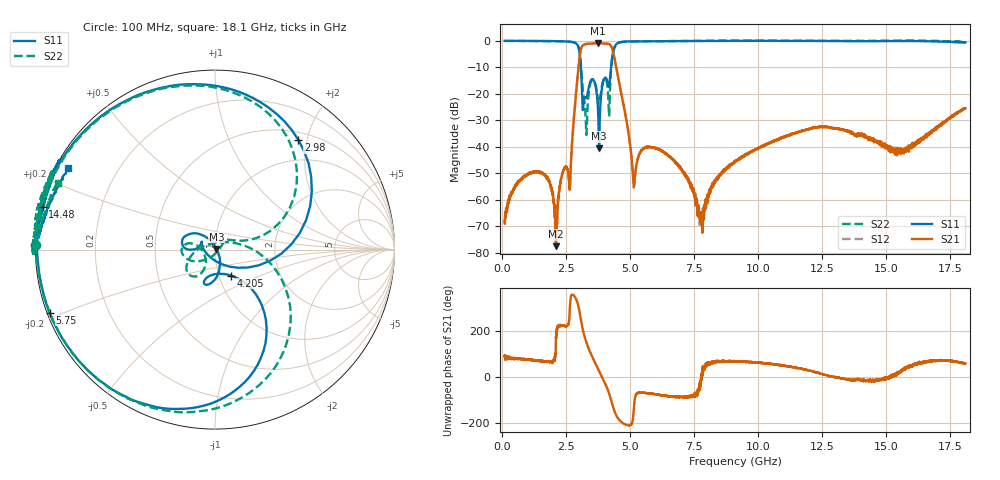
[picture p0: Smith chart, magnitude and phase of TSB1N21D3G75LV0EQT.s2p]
! TSB1N21D3G75LV0EQT  S-PARAMETER MODEL  ( General Type )
! Model Generated by TAIYO YUDEN Corporation (https://www.yuden.co.jp/en/)
! Version 1.0
! TAIYO YUDEN Control No. 20240527
! Copyright(c) 2024 TAIYO YUDEN CO.,LTD. All Rights Reserved.
! Products Name : Ceramic RF Devices
! Characteristics :
!  Passband freq : 3300-4200MHz ( At Passband , Insertion Loss : 2.0dB , VSWR 2.0 ),
!  Attenuation : 35 dB min at 600 to 2700MHz, 20 dB min at 4900 to 5900MHz, Impedance : 50 Ohm ,
!  Case Size : 2 x 1.25 / 0.079 x 0.049 [mm/inch] , Thickness : 0.65/ 0.026 [mm/inch]
!  (Conditions: Temperature = 25 degC , DC Bias Current/Voltage = 0A / 0V)
! External Node Assignments :
!  1  o---|-------|---o  2
!  |  BPF  |
! GND o---|-------|---o GND
! Frequency Range : 100MHz  -  18.1GHz  [ 3601 STEP ]
# MHZ S RI R 50
! Freq[MHz].  S11 Real  S11 Imag  S21 Real  S21 Imag  S12 Real  S12 Imag  S22 Real  S22 Imag
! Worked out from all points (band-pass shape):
!   3601 points, 100 MHz to 18.1 GHz, reference 50 ohm
!   highest |S21| = -0.80 dB at 3.755 GHz (marker M1); lowest = -77.6 dB at 2.105 GHz (marker M2)
!   |S21| within 3 dB of the highest: 3.069 GHz to 4.326 GHz (1.258 GHz wide, 34 % of centre)
!   lowest |S11| = -40.6 dB at 3.79 GHz (marker M3), VSWR 1.02, Z = 50.8 + j0.418 ohm
!   |S11| at or under -10 dB: 3.079 GHz to 4.255 GHz (1.176 GHz wide, 32.1 % of centre)
!   |S22| runs from -35.6 to 0.2 dB; largest |S21 - S12| = 0.0036
!   S11 on the Smith chart (normalised r, x): 100 MHz: -0.00, +0.01; 2.98 GHz: 0.62, +1.85; 4.205 GHz: 1.14, -0.34; 5.75 GHz: 0.01, -0.18; 14.48 GHz: 0.01, +0.12; 18.1 GHz: 0.04, +0.26
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100  -1.001 0.0239  -1.71e-06 0.000384  7.33e-05 0.000373  -0.9975 0.0244
1360  -0.9507 0.2975  0.00103 0.00315  0.00102 0.00318  -0.9471 0.2932
2105  -0.8359 0.5301  -0.000132 7.2e-06  -0.000195 7.2e-05  -0.8405 0.5139
2365  -0.7336 0.6551  -0.00225 -0.0023  -0.00224 -0.00226  -0.7472 0.6329
2650  -0.4868 0.8342  0.000983 -0.00133  0.000871 -0.00136  -0.526 0.8078
2980  0.4647 0.6114  0.1941 -0.2235  0.194 -0.2234  0.3388 0.7161
3100  0.1846 -0.0996  -0.3874 -0.628  -0.387 -0.6282  0.2688 0.0803
3260  -0.0725 0.0428  -0.8324 0.2452  -0.8326 0.2453  0.0353 0.0191
3435  -0.1618 0.00448  -0.306 0.8343  -0.3054 0.8343  -0.1345 -0.0622
3755  -0.0143 0.0391  0.7514 0.5172  0.7512 0.5167  -0.0739 -0.00109
3790  0.00833 0.00411  0.8158 0.4069  0.8159 0.4068  -0.0595 -0.0283
4205  0.089 -0.1446  0.1427 -0.847  0.1426 -0.8464  0.0688 0.0411
4520  -0.1974 -0.8875  -0.2228 -0.000711  -0.2227 -0.000543  -0.0562 -0.8968
5140  -0.7941 -0.5773  -0.00187 -0.0008  -0.00178 -0.000822  -0.7515 -0.628
5750  -0.921 -0.3506  0.00281 -0.00943  0.00283 -0.0094  -0.9029 -0.3932
6100  -0.9545 -0.2518  0.00181 -0.00887  0.00186 -0.00897  -0.9448 -0.2902
7795  -0.9914 0.0971  0.000416 0.000118  0.000537 -2.87e-05  -1.002 0.0552
9100  -0.9654 0.2796  0.00194 0.00487  0.00217 0.00483  -0.9946 0.2025
12100  -0.866 0.4939  0.0203 0.00953  0.0199 0.00962  -0.908 0.4331
14485  -0.9597 0.2392  0.0134 -0.00345  0.0134 -0.00389  -0.9798 0.2065
15100  -0.9799 0.1573  0.0101 -0.000436  0.0101 -0.00063  -1.002 0.1093
18100  -0.8163 0.4547  0.0283 0.0453  0.029 0.0463  -0.8767 0.3712
